//{{V2}}
FUNCTION FC16
TITLE=Write UInt32 SDO
//*****************************************************************************
//* maxon motor ag
//* R&D
//* all rights reserved
//*****************************************************************************
//* Summary:  Write an UInt32 object via SDO
//*
//* Remarks:
//*
//* Created under: STEP7 REV5.2+SP1
//*****************************************************************************
//* History:
//* 18.05.2004 | INA   first release
//*
//*
//*****************************************************************************


AUTHOR:INA
FAMILY:SDO
NAME:WrUInt32
VERSION:00.01


VAR_INPUT
       NodeID:BYTE
       Index:DWORD
       SubIndex:DWORD
       ValueIn:DWORD
END_VAR

VAR_OUTPUT
       RET_VAL:BOOL //Done
       Err:BOOL //True = Error detected
       ErrNo:DINT //Error number (CAN or/and VIPA!)
END_VAR

VAR_IN_OUT
END_VAR

VAR_TEMP
       xBusy:BOOL //The write job is not yet completed
       xCanOpenError:DWORD //Return value from SDO transfer
       xRetValue:WORD //VIPA Error
       xValueIn:DWORD
END_VAR
BEGIN

NETWORK
TITLE=
//{{a}}

// SDO Write UInt32

       R    #RET_VAL                     // Done
       R    #Err
       L    0
       T    #ErrNo

       L    #ValueIn
       T    #xValueIn

sfc   :NOP  0

       CALL SFC219
         Request:=TRUE
         Slot_Master:=B#16#00
         NodeID:=#NodeID
         Transfertyp:=B#16#23            // Write
         Index:=#Index
         Subindex:=#SubIndex
         CanOpenError:=#xCanOpenError
         RetVal:=#xRetValue
         Busy:=#xBusy
         DataBuffer:=P#L 8.0 DWORD 1

       L    1
       U    #xBusy
       SPB  sfc

       S    #RET_VAL

       L    W#16#F021
       L    #xRetValue
       <I
       SPB  ok                           // jump if RetValue lower than 0xF021
       L    W#16#F028
       L    #xRetValue
       >I
       SPBN errV                         // jump if xRetValue between 0xF021 and 0xF028

       L    0
       L    #xCanOpenError
       <>D
       SPB  errC                         // jump if CAN error

ok    :NOP  0
       R    #Err
       SPA  end

errC  :NOP  0                            // CANopen error
       S    #Err
       L    #xCanOpenError
       TAD
       T    #ErrNo
       SPA  end

errV  :NOP  0                            // VIPA error
       S    #Err
       L    0
       T    #ErrNo
       L    #xRetValue                   // RetVal
       T    #ErrNo

end   :NOP  0
END_FUNCTION
